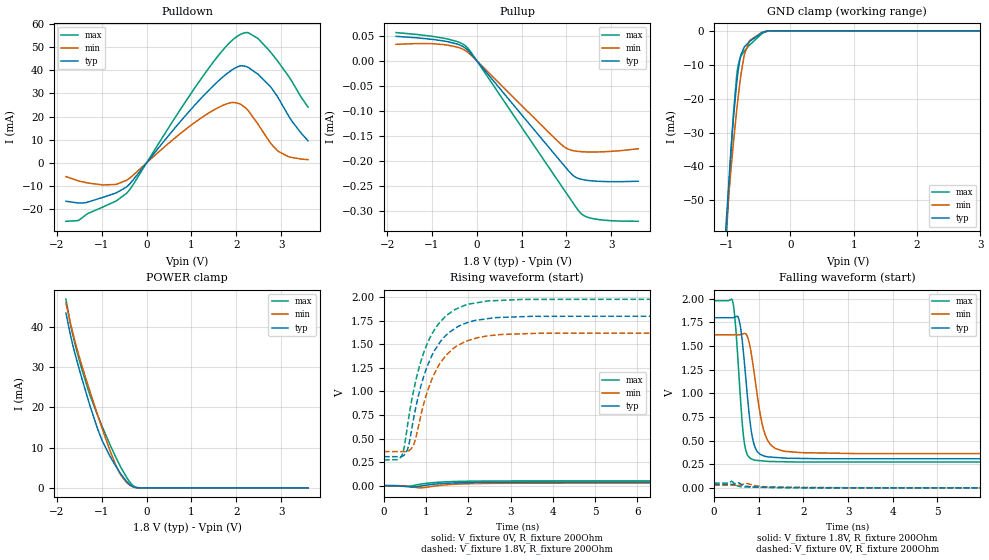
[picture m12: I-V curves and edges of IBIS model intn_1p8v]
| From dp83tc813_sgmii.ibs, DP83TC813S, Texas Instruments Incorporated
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| intn_1p8v
[Model]   intn_1p8v
Model_type   Output
Polarity   Non-Inverting
Vmeas = 0.9
Vref = 0.9
Cref = 2pF
Rref = 100000
|   typ   min   max
C_comp   2.12pF   2.14pF   2.1pF
[Voltage Range]   1.8   1.62   1.98
[Temperature Range]   27   150   -40
[Pullup Reference]   1.8   1.62   1.98
[Pulldown Reference]   0   0   0
[Power Clamp Reference]   1.8   1.62   1.98
[GND Clamp Reference]   0   0   0
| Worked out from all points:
|   slope of the pulldown table from 0 to 0.27 V, typ, clamps not added: 41.1 ohm
|   slope of the pullup table from 0 to 0.27 V, typ, clamps not added: 9.25 kohm
|   GND clamp passes 1 mA (typ) near -0.48 V on its own axis
|   POWER clamp passes 1 mA (typ) near -0.39 V on its own axis
|   falling waveform, V_fixture 1.8V, R_fixture 200Ohm: 20-80 % time 189ps typ, 260ps min, 151ps max; typ from 1.8 V to 0.307 V
|   rising waveform, V_fixture 1.8V, R_fixture 200Ohm: 20-80 % time 635ps typ, 636ps min, 625ps max; typ from 0.307 V to 1.8 V
[Pulldown]
|   Voltage   I(typ)   I(min)   I(max)
-1.8V     -16.61mA   -5.947mA   -25.29mA
-1.53V    -17.36mA   -7.777mA   -25mA
-973.8mV  -14.92mA   -9.557mA   -19.1mA
-444.6mV  -10.39mA   -7.539mA   -13.15mA
1.294V    29.56mA    20.41mA    38.51mA
1.823V    39.07mA    25.75mA    51.41mA
2.099V    41.94mA    25.27mA    55.59mA
2.266V    41.26mA    22.56mA    56.3mA
2.477V    38.44mA    16.93mA    53.86mA
2.936V    28.08mA    4.971mA    43.64mA
3.249V    17.82mA    2.251mA    34.94mA
3.6V      9.489mA    1.359mA    24.09mA
[GND Clamp]
|   Voltage   I(typ)   I(min)   I(max)
-1.8V     -336.1mA   -294mA     -377.2mA
-1.044V   -67.3mA    -66.5mA    -74.32mA
-1.006V   -55.59mA   -57.15mA   -60.5mA
-946.8mV  -38.53mA   -43.59mA   -40.01mA
-892.8mV  -25.18mA   -32.5mA    -23.85mA
-844.2mV  -15.46mA   -23.5mA    -13.26mA
-822.6mV  -12.02mA   -19.84mA   -10.34mA
-774mV    -6.89mA    -12.58mA   -7.326mA
-720mV    -4.668mA   -6.753mA   -5.905mA
-639mV    -3.109mA   -2.848mA   -4.151mA
-444.6mV  -532.9uA   -446.3uA   -818uA
3.6V      0A         0A         0A
[Pullup]
|   Voltage   I(typ)   I(min)   I(max)
-1.8V     48.62uA    32.67uA    56.18uA
-957.6mV  42.23uA    33.83uA    48.18uA
-444.6mV  33.54uA    27.37uA    38.45uA
-261mV    25.56uA    20.53uA    30.29uA
-120.6mV  12.95uA    10.59uA    15.91uA
1.894V    -203.6uA   -168uA     -250.6uA
1.975V    -212.2uA   -173.5uA   -261.3uA
2.131V    -227.8uA   -179.2uA   -281.8uA
2.331V    -236.8uA   -181.7uA   -305.7uA
2.477V    -239.1uA   -182.2uA   -312.8uA
2.709V    -240.8uA   -182.2uA   -317.1uA
3.6V      -240.7uA   -175.9uA   -320.7uA
[POWER Clamp]
|   Voltage   I(typ)   I(min)   I(max)
-1.8V     43.38mA    45.82mA    46.84mA
-1.681V   37.05mA    40.07mA    39.68mA
-1.508V   29.65mA    32.74mA    31.93mA
-1.292V   21.44mA    24.91mA    23.94mA
-1.082V   14.27mA    17.71mA    17.68mA
-963mV    11.04mA    13.8mA     14.48mA
-822.6mV  7.958mA    9.405mA    10.86mA
-617.4mV  4.151mA    3.997mA    6.014mA
-444.6mV  1.573mA    1.284mA    2.566mA
-293.4mV  232.3uA    227.3uA    490.3uA
-136.8mV  3.538uA    9.732uA    5.794uA
3.6V      0A         0A         0A
[Ramp]
R_load = 200
|   typ   min   max
dV/dt_r   0.0226246/7.07366e-10  0.0167793/7.93702e-10  0.0306174/6.69136e-10
dV/dt_f   0.895548/1.89087e-10   0.754967/2.59549e-10   1.02397/1.5047e-10
[Falling Waveform]
V_fixture = 1.8V
V_fixture_min = 1.62V
V_fixture_max = 1.98V
R_fixture = 200Ohm
C_fixture = 0F
|   Time   V(typ)   V(min)   V(max)
0s        1.8V       1.62V      1.98V
403.4ps   1.8V       1.62V      1.99V
468.5ps   1.808V     1.62V      1.779V
550.3ps   1.792V     1.62V      1.233V
687.1ps   1.278V     1.635V     446.3mV
793.9ps   741.8mV    1.516V     319.6mV
886.7ps   473mV      1.25V      296mV
1.154ns   332.1mV    548.8mV    282.1mV
1.557ns   316mV      389.3mV    276.3mV
12ns      307.4mV    361.7mV    273.4mV
[Rising Waveform]
V_fixture = 0V
V_fixture_min = 0V
V_fixture_max = 0V
R_fixture = 200Ohm
C_fixture = 0F
|   Time   V(typ)   V(min)   V(max)
0s        467.9nV    8.454uV    175.3nV
330.9ps   -569.6uV   -207.8uV   -3.154mV
558.4ps   -9.633mV   -6.988mV   -8.05mV
688.2ps   -14.98mV   -15.01mV   1.122mV
874.1ps   -3.632mV   -23.2mV    16.53mV
1.128ns   12.93mV    -8.761mV   30.6mV
1.404ns   23.44mV    6.465mV    39.61mV
1.762ns   30.32mV    17.05mV    45.2mV
2.18ns    34.01mV    22.4mV     48.3mV
12ns      37.71mV    27.97mV    51.03mV
[Rising Waveform]
V_fixture = 1.8V
V_fixture_min = 1.62V
V_fixture_max = 1.98V
R_fixture = 200Ohm
C_fixture = 0F
|   Time   V(typ)   V(min)   V(max)
0s        307.4mV    361.7mV    273.4mV
418.7ps   310.4mV    361.4mV    315mV
558.9ps   384.7mV    365.8mV    642.5mV
657.6ps   599.6mV    398.5mV    905.7mV
869.7ps   1.049V     736.8mV    1.313V
1.138ns   1.383V     1.134V     1.613V
1.475ns   1.598V     1.386V     1.805V
1.909ns   1.72V      1.526V     1.913V
3.671ns   1.798V     1.618V     1.977V
12ns      1.8V       1.62V      1.98V
[Falling Waveform]
|Gnd
V_fixture = 0V
V_fixture_min = 0V
V_fixture_max = 0V
R_fixture = 200Ohm
C_fixture = 0F
|   Time   V(typ)   V(min)   V(max)
0s        37.71mV    27.97mV    51.03mV
323.3ps   37.31mV    27.48mV    50.79mV
394.5ps   37.5mV     27.62mV    68.91mV
517.8ps   55.97mV    27.86mV    22.34mV
594.2ps   41.97mV    28.95mV    13.09mV
697.7ps   19.98mV    45.38mV    9.746mV
810.4ps   11.7mV     37.1mV     8.114mV
1.053ns   7.754mV    14.15mV    5.219mV
1.507ns   4.563mV    7.521mV    1.031mV
12ns      505.7nV    8.487uV    159.8nV
